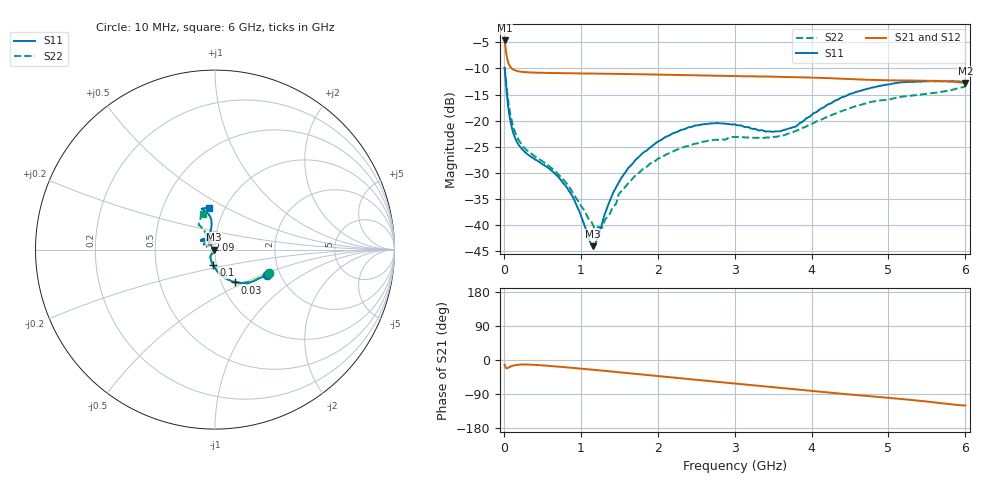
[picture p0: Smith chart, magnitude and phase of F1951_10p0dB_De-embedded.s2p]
! Integrated Device Technology
! Corporate Headquarters
! 6024 Silver Creek Valley Road
! San Jose, CA 95138  USA
! Phone:  1-408-284-8200
! Toll Free:  1-800-223-1366
! Webpage:  http://www.idt.com/
! Timing and RF Division
! 515 Groton Road, Suite 102
! Westford, MA 01886-6024
! Device:  F1951
! Description: 6-bit 0.5 dB Digital Step Attenuator
! Frequency:  100.0 -  4000.00 MHz
! Package:  4x4 mm Thin QFN Plastic Package: 24 pin
! Ports:  2 RF, 6 DC
!  Pin  1  = NC
!  Pin  2  = RF1  =  Port 1
!  Pin  3  = GND
!  Pin  4  = NC
!  Pin  5  = Serial Data Out (SDO)
!  Pin  6  = NC
!  Pin  7  = Reset Bar ( RSTb)
!  Pin  8  = Clock (CLK)
!  Pin  9  = Chip Select Bar (CSb)
!  Pin 10  = NC
!  Pin 11  = Serial Data In (SDI)
!  Pin 12  = NC
!  Pin 13  = NC
!  Pin 14  = VDD
!  Pin 15  = NC
!  Pin 16  = GND
!  Pin 17  = RF2  =  Port 2
!  Pin 18  = NC
!  Pin 19  = GND
!  Pin 20  = GND
!  Pin 21  = GND
!  Pin 22  = GND
!  Pin 23  = GND
!  Pin 24  = GND
! State:  20
! Atten State:  10.0 dB
! Voltage:  +3.30 Volts
! Current:  0.475 mA
! Data:  The device was measured on a F195X evaluation board which has
!  individual transmission lines to the RF pins.  Data was collected
!  de-embedded using a Automatic Fixture Removal [AFR] (Keysight Technologies).
!  The reference plane is the edge of the package pin.
! Misc:  Lot Code  1225BCA
!  Action Tracker AT0399
! Date Measured:  2018-09-13
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# GHz S dB R 50
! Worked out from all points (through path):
!   600 points, 10 MHz to 6 GHz, reference 50 ohm
!   highest |S21| = -4.65 dB at 10 MHz (marker M1); lowest = -12.8 dB at 6 GHz (marker M2)
!   group delay of S21, straight-line fit = 52.6 ps
!   lowest |S11| = -44.0 dB at 1.16 GHz (marker M3), VSWR 1.01, Z = 49.4 + j0.0266 ohm
!   |S11| at or under -10 dB: 10.7 MHz to end of sweep
!   |S22| runs from -40.6 to -9.7 dB; largest |S21 - S12| = 0.0005
!   S11 on the Smith chart (normalised r, x): 10 MHz: 1.70, -0.54; 30 MHz: 1.16, -0.44; 100 MHz: 0.97, -0.17; 2.09 GHz: 0.91, +0.10; 6 GHz: 0.84, +0.41
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0.01  -9.88 -26.3  -4.65 -12.3  -4.65 -12.3  -9.75 -23.4
0.03  -13.43 -59.1  -6.98 -21.7  -6.98 -21.7  -12.74 -53.4
0.06  -17.69 -81.0  -8.99 -20.1  -9.00 -20.1  -16.59 -75.9
0.1  -21.10 -95.9  -9.96 -16.1  -9.97 -16.1  -19.88 -91.8
0.16  -23.75 -109.0  -10.44 -13.2  -10.44 -13.2  -22.71 -105.5
0.25  -25.64 -118.7  -10.67 -12.0  -10.67 -11.9  -24.91 -116.7
0.71  -30.76 -123.1  -10.90 -17.4  -10.89 -17.5  -30.28 -127.3
0.88  -34.15 -123.6  -10.94 -20.5  -10.94 -20.5  -33.36 -129.0
1.01  -38.46 -129.9  -10.97 -22.9  -10.97 -22.9  -36.45 -133.8
1.16  -43.98 177.6  -10.99 -25.7  -10.99 -25.7  -40.03 -158.2
1.27  -40.00 128.7  -11.00 -27.8  -11.01 -27.8  -40.53 167.7
1.4  -34.50 114.3  -11.03 -30.4  -11.03 -30.4  -37.06 139.6
1.53  -30.88 113.4  -11.06 -32.8  -11.06 -32.8  -33.45 130.5
2.01  -23.92 125.0  -11.18 -42.5  -11.18 -42.5  -27.20 134.4
2.09  -23.21 127.0  -11.20 -44.1  -11.20 -44.1  -26.64 136.2
2.5  -20.89 139.5  -11.32 -52.3  -11.32 -52.3  -24.36 147.8
3.01  -20.74 148.1  -11.47 -62.3  -11.47 -62.2  -23.08 153.5
3.58  -22.03 125.4  -11.59 -73.4  -11.59 -73.5  -22.91 135.5
4.01  -18.78 101.1  -11.75 -81.9  -11.75 -81.9  -20.58 121.8
4.49  -14.94 97.9  -12.02 -90.9  -12.02 -90.9  -17.63 120.3
5.01  -13.04 105.2  -12.28 -100.0  -12.28 -100.0  -15.95 123.0
6  -12.68 98.9  -12.78 -120.2  -12.78 -120.2  -13.45 109.0
